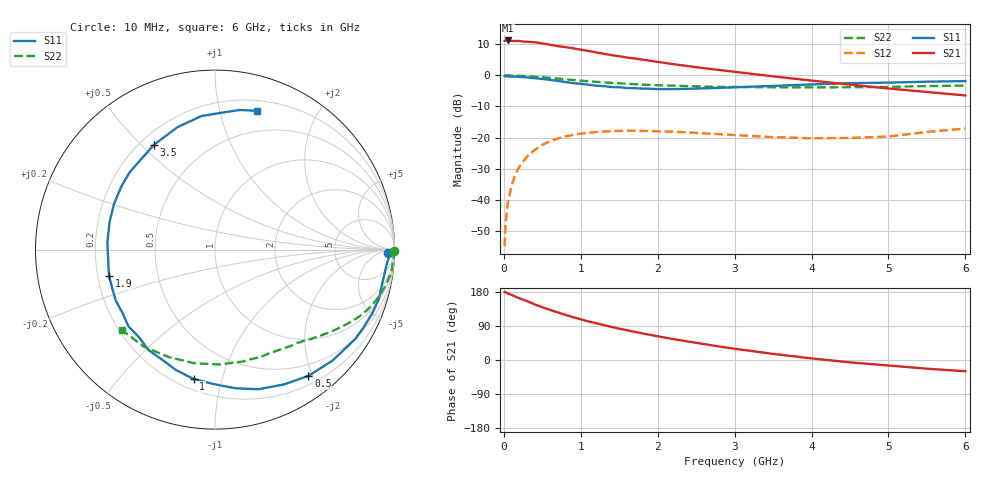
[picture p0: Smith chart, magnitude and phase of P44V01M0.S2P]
! SIEMENS Small Signal Semiconductors
! BFP182
! Si NPN RF Bipolar Junction Transistor in SOT143
! VCE = 4 V  IC = 1 mA
! Common Emitter S-Parameters:  March  1996
# GHz  S  MA  R  50
!  f  S11  S21  S12  S22
! GHz  MAG  ANG  MAG  ANG  MAG  ANG  MAG  ANG
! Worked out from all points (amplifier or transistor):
!   36 points, 10 MHz to 6 GHz, reference 50 ohm
!   highest |S21| = 11.2 dB at 50 MHz (marker M1)
!   |S21| within 3 dB of that: start of sweep to 1.007 GHz
!   unconditionally stable (mu >= 1): 2.627 GHz to end of sweep
!   at 250 MHz: K = 0.10, MSG = 19.3 dB, |S12| = -27.7 dB
!   at 1.4 GHz: K = 0.54, MSG = 12.2 dB, |S12| = -17.9 dB
!   at 6 GHz: K = 1.08, MAG = 3.5 dB, |S12| = -17.1 dB
!   S11 on the Smith chart (normalised r, x): 10 MHz: 45, -22; 500 MHz: 0.32, -1.94; 1 GHz: 0.26, -0.81; 1.9 GHz: 0.25, -0.11; 3.5 GHz: 0.25, +0.55; 6 GHz: 0.29, +1.30
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0.01  0.965 -1.0  3.583 179.6  0.0018 85.3  0.9987 -0.3
0.02  0.97 -2.3  3.597 179.0  0.0037 95.2  0.9936 -0.8
0.05  0.9587 -5.4  3.63 175.9  0.0088 87.1  0.9978 -2.0
0.1  0.9512 -11.0  3.571 171.7  0.0168 81.6  0.992 -4.1
0.2  0.9457 -22.0  3.574 163.1  0.0338 76.2  0.9867 -8.1
0.4  0.9006 -43.4  3.395 146.9  0.0633 63.5  0.9529 -15.5
0.5  0.8752 -53.5  3.255 139.2  0.0761 57.3  0.9312 -19.0
0.6  0.8436 -63.0  3.105 132.4  0.0876 51.6  0.9089 -22.1
0.8  0.7807 -81.6  2.838 119.1  0.1041 41.9  0.8634 -27.4
0.9  0.7487 -90.8  2.721 113.0  0.1107 37.2  0.8411 -29.7
1  0.7305 -99.4  2.578 107.4  0.1154 33.0  0.8204 -32.0
1.1  0.7055 -107.9  2.47 101.7  0.1196 29.4  0.8023 -34.0
1.3  0.6711 -123.5  2.218 92.2  0.1249 22.7  0.7699 -37.7
1.5  0.6447 -138.4  2.028 82.7  0.1277 17.2  0.7433 -41.0
1.9  0.6082 -166.1  1.716 66.4  0.1272 8.5  0.701 -47.4
2.2  0.6008 176.1  1.511 55.2  0.1241 4.0  0.6821 -52.1
2.8  0.6291 146.1  1.216 35.6  0.1134 -1.6  0.6518 -62.3
3.5  0.6758 120.3  0.963 16.1  0.1016 -1.8  0.6421 -76.3
4  0.7135 107.0  0.823 4.2  0.0974 2.6  0.6405 -87.9
4.5  0.7476 95.9  0.709 -6.2  0.0986 7.7  0.6435 -100.3
5.5  0.7898 80.0  0.54 -22.9  0.1232 16.8  0.6706 -126.2
6  0.8074 73.3  0.474 -29.7  0.1398 15.6  0.6849 -139.0
